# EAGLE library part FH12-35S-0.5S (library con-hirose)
0.5mm Pitch Connectors For FPC/FFC Source: Data sheet
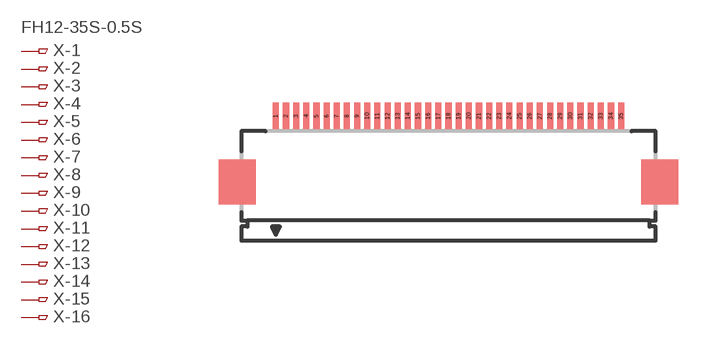
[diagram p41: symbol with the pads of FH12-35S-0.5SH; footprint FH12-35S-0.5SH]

Designator prefix X; gates -1=PINV -2=PIN -3=PIN -4=PIN -5=PIN -6=PIN -7=PIN -8=PIN -9=PIN -10=PIN -11=PIN -12=PIN -13=PIN -14=PIN -15=PIN -16=PIN -17=PIN -18=PIN -19=PIN -20=PIN -21=PIN -22=PIN -23=PIN -24=PIN -25=PIN -26=PIN -27=PIN -28=PIN -29=PIN -30=PIN -31=PIN -32=PIN -33=PIN -34=PIN -35=PIN

## FH12-35S-0.5SH (OC_FARNELL: unknown; OC_NEWARK: unknown)  [FH12-35S-0.5SH]
1  -1:1  pas
2  -2:1  pas
3  -3:1  pas
4  -4:1  pas
5  -5:1  pas
6  -6:1  pas
7  -7:1  pas
8  -8:1  pas
9  -9:1  pas
10  -10:1  pas
11  -11:1  pas
12  -12:1  pas
13  -13:1  pas
14  -14:1  pas
15  -15:1  pas
16  -16:1  pas
17  -17:1  pas
18  -18:1  pas
19  -19:1  pas
20  -20:1  pas
21  -21:1  pas
22  -22:1  pas
23  -23:1  pas
24  -24:1  pas
25  -25:1  pas
26  -26:1  pas
27  -27:1  pas
28  -28:1  pas
29  -29:1  pas
30  -30:1  pas
31  -31:1  pas
32  -32:1  pas
33  -33:1  pas
34  -34:1  pas
35  -35:1  pas

## Footprint FH12-35S-0.5SH (pad centres in mm)
0.5mm Pitch Connectors For FPC/FFC Source: Data sheet
smd 0.3 x 1.3: 1 -8.5,3.25; 2 -8,3.25; 3 -7.5,3.25; 4 -7,3.25; 5 -6.5,3.25; 6 -6,3.25; 7 -5.5,3.25; 8 -5,3.25; 9 -4.5,3.25; 10 -4,3.25; 11 -3.5,3.25; 12 -3,3.25; 13 -2.5,3.25; 14 -2,3.25; 15 -1.5,3.25; 16 -1,3.25; 17 -0.5,3.25; 18 0,3.25; 19 0.5,3.25; 20 1,3.25; 21 1.5,3.25; 22 2,3.25; 23 2.5,3.25; 24 3,3.25; 25 3.5,3.25; 26 4,3.25; 27 4.5,3.25; 28 5,3.25; 29 5.5,3.25; 30 6,3.25; 31 6.5,3.25; 32 7,3.25; 33 7.5,3.25; 34 8,3.25; 35 8.5,3.25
